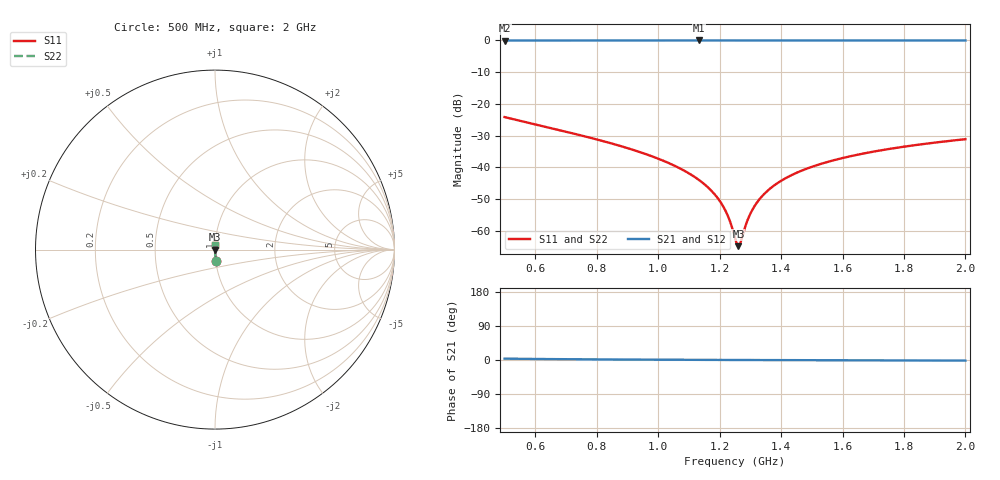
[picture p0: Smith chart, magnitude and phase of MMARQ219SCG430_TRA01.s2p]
! MMARQ219SCG430_TRA01  S-PARAMETER MODEL  ( General Type )
! Model Generated by TAIYO YUDEN Corporation (http://www.ty-top.com)
! Version 1.0
! TAIYO YUDEN Control No. 180601
! Copyright(c) 2018 TAIYO YUDEN CO.,LTD. All Rights Reserved.
! Product Description (link to TY-COMPAS)
! https://ds.yuden.co.jp/TYCOMPAS/or/detail?pn=MMARQ219SCG430JTRA01&u=M
! Products Name : Multilayer Ceramic Capacitors
! Characteristics :
!  Capacitance : 43 pF , Rated Voltage : 250V , TCC : CG / C0G
!  Case Size : 2.0 x 1.25 / 0.079 x 0.049 [mm/inch] , Thickness : 0.85 / 0.033 [mm/inch]
!  (Conditions: Temperature = 25 degC , DC Bias Current/Voltage = 0A / 0V)
! External Node Assignments :
!  1  o---| |---o  2
! GND o---------o GND
! Frequency Range : 500MHz  -  2000MHz  [ 401 STEP ]
# MHz S RI R 50
! Freq[MHz].  S11 Real  S11 Imag  S21 Real  S21 Imag  S12 Real  S12 Imag  S22 Real  S22 Imag
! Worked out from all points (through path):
!   401 points, 500 MHz to 2 GHz, reference 50 ohm
!   highest |S21| = 0.00 dB at 1.134 GHz (marker M1); lowest = 0.0 dB at 500 MHz (marker M2)
!   lowest |S11| = -64.9 dB at 1.261 GHz (marker M3), VSWR 1.00, Z = 50.1 - j0.000451 ohm
!   |S11| at or under -10 dB: start of sweep to end of sweep
!   |S22| runs from -64.9 to -24.2 dB; largest |S21 - S12| = 0
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500  0.00418 -0.0616  0.9958 0.0616  0.9958 0.0616  0.00418 -0.0616
751.25  0.00141 -0.0315  0.9986 0.0315  0.9986 0.0315  0.00141 -0.0315
893.75  0.00087 -0.0204  0.9991 0.0204  0.9991 0.0204  0.00087 -0.0204
1002.5  0.000665 -0.0135  0.9993 0.0135  0.9993 0.0135  0.000665 -0.0135
1077.5  0.000591 -0.00919  0.9994 0.00919  0.9994 0.00919  0.000591 -0.00919
1133.75  0.000563 -0.00621  0.9994 0.00621  0.9994 0.00621  0.000563 -0.00621
1175  0.000555 -0.00412  0.9994 0.00412  0.9994 0.00412  0.000555 -0.00412
1205  0.000555 -0.00266  0.9994 0.00266  0.9994 0.00266  0.000555 -0.00266
1227.5  0.000558 -0.00158  0.9994 0.00158  0.9994 0.00158  0.000558 -0.00158
1250  0.000564 -0.000525  0.9994 0.000525  0.9994 0.000525  0.000564 -0.000525
1257.5  0.000566 -0.000177  0.9994 0.000177  0.9994 0.000177  0.000566 -0.000177
1261.25  0.000567 -4.5e-06  0.9994 4.5e-06  0.9994 4.5e-06  0.000567 -4.5e-06
1268.75  0.00057 0.00034  0.9994 -0.00034  0.9994 -0.00034  0.00057 0.00034
1287.5  0.000578 0.00119  0.9994 -0.00119  0.9994 -0.00119  0.000578 0.00119
1302.5  0.000586 0.00186  0.9994 -0.00186  0.9994 -0.00186  0.000586 0.00186
1321.25  0.000596 0.00269  0.9994 -0.00269  0.9994 -0.00269  0.000596 0.00269
1343.75  0.000611 0.00368  0.9994 -0.00368  0.9994 -0.00368  0.000611 0.00368
1407.5  0.000662 0.00637  0.9993 -0.00637  0.9993 -0.00637  0.000662 0.00637
1501.25  0.000761 0.0102  0.9992 -0.0102  0.9992 -0.0102  0.000761 0.0102
1610  0.000906 0.0143  0.9991 -0.0143  0.9991 -0.0143  0.000906 0.0143
1752.5  0.00114 0.0194  0.9989 -0.0194  0.9989 -0.0194  0.00114 0.0194
2000  0.00164 0.0276  0.9984 -0.0276  0.9984 -0.0276  0.00164 0.0276
